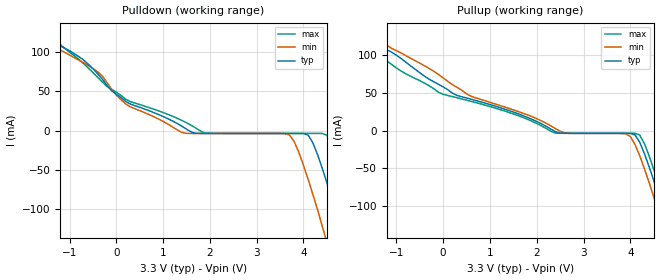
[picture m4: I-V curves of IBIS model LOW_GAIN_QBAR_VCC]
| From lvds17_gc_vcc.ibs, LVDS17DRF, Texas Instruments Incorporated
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|   Q_bar Output Model
[Model]   LOW_GAIN_QBAR_VCC
Model_type   Output_ECL
| Signals   Q/
Vmeas = 2.0V   |Reference voltage for timing measurements
Cref = 0pF   |Timing specification test load capacitance value
| variable   typ   min   max
C_comp   0.6pF   0.4pF   0.7pF
|   typ   min   max
[Temperature Range]   25   -40   85
[Voltage range]   3.3V   3.0V   3.6V
[Pulldown]
|Voltage I(typ)   I(min)   I(max)
| Note that the[Pulldown]voltage table for (P)ECL is referenced
| to Vcc and is calculated using Vtable=Vcc - Vmeasured.
-3.3V     261mA      264mA      257mA
-1.9V     132mA      131mA      137mA
-400mV    72.6mA     75mA       68.1mA
200mV     37.2mA     34mA       39.9mA
1.4V      5.56mA     -2.38mA    12.9mA
1.9V      -3.69mA    -3.75mA    -3.34mA
3.7V      -3.75mA    -5.66mA    -3.64mA
4.1V      -5.83mA    -62.5mA    -3.65mA
4.5V      -66.6mA    -143mA     -5.94mA
4.8V      -127mA     -208mA     -51.6mA
5.2V      -214mA     -300mA     -132mA
6.6V      -556mA     -653mA     -461mA
[Pullup]
|Voltage   I(typ)   I(min)   I(max)
| Note that the[Pullup]voltage table is referenced to Vcc
| and is calculated using Vtable=Vcc - Vmeasured.
-3.3V     260mA      298mA      226mA
-2.3V     161mA      199mA      140mA
-1.7V     124mA      143mA      116mA
-100mV    61.4mA     74.4mA     50.8mA
600mV     41.5mA     45.4mA     38.7mA
2.4V      -1.58mA    2.54mA     -3.42mA
3.9V      -3.75mA    -4.27mA    -3.65mA
4.2V      -15.6mA    -33.5mA    -5.94mA
4.7V      -106mA     -129mA     -90.8mA
4.9V      -148mA     -171mA     -132mA
5V        -170mA     -193mA     -154mA
6.6V      -556mA     -581mA     -538mA
[Ramp]
|   typ   min   max
dV/dt_r   0.460/252ps   0.459/262ps   0.459/220ps
dV/dt_f   0.460/219ps   0.459/249ps   0.459/202ps
